ORGANIZATION_BLOCK "Hardware Interrupt 1"
TITLE =
VERSION : 0.1


VAR_TEMP
  OB41_EV_CLASS : BYTE ;	//Bits 0-3 = 1 (Coming event), Bits 4-7 = 1 (Event class 1)
  OB41_STRT_INF : BYTE ;	//16#41/42/43/44 (Interrupt 1/2/3/4)
  OB41_PRIORITY : BYTE ;	//17 (Priority of 1 is lowest)
  OB41_OB_NUMBR : BYTE ;	//41 (Organization block 41, OB41)
  OB41_RESERVED_1 : BYTE ;	//Reserved for system
  OB41_RESERVED_2 : BYTE ;	//Reserved for system
  OB41_MDL_ADDR : WORD ;	//Base address of module initiating interrupt
  OB41_POINT_ADDR : DWORD ;	//Address of interrupt point on module
  OB41_DATE_TIME : DATE_AND_TIME ;	//Date and time OB41 started
END_VAR
BEGIN
END_ORGANIZATION_BLOCK

